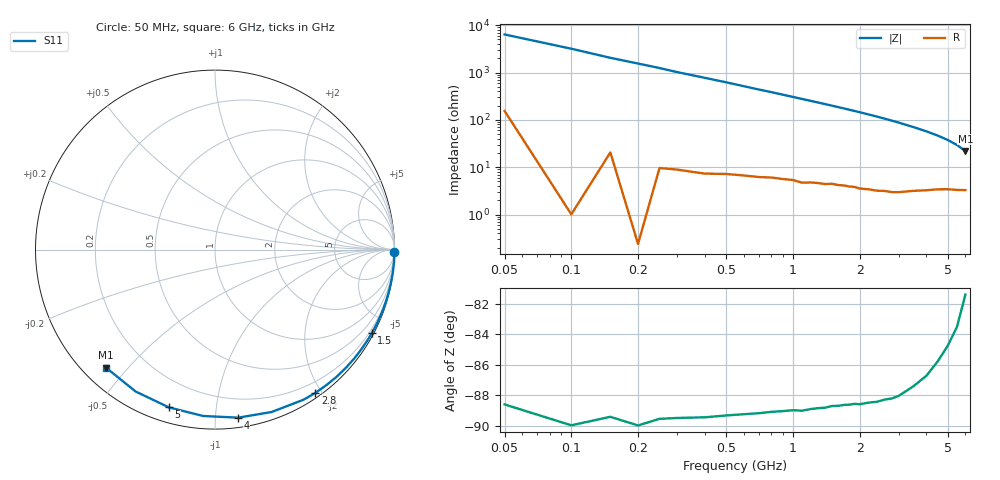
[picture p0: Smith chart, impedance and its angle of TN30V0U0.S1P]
! SIEMENS Discrete & RF Semiconductors
! BAS70-07W
! Si Schottky Diode in SOT343
! VR = 30 V
! S-Parameters:  February  1997
# GHz  S  MA  R  50
!  f  S11
! GHz  MAG  ANG
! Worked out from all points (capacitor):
!   34 points, 50 MHz to 6 GHz, reference 50 ohm
!   read as one part to ground: C = 500 fF near 50 MHz
!   lowest |Z| = 22 ohm at 6 GHz (marker M1)
!   S11 on the Smith chart (normalised r, x): 50 MHz: open; 1.5 GHz: 0.09, -3.99; 2.8 GHz: 0.06, -1.92; 4 GHz: 0.07, -1.14; 5 GHz: 0.07, -0.75; 6 GHz: 0.07, -0.44
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0.05  0.9996 -0.9
0.2  1 -3.7
0.25  0.9994 -4.6
0.3  0.9991 -5.6
0.4  0.9988 -7.4
0.6  0.9975 -11.1
0.7  0.9968 -13.0
0.8  0.996 -14.8
0.9  0.9953 -16.7
1.1  0.994 -20.5
1.3  0.9918 -24.3
1.4  0.991 -26.2
1.5  0.9895 -28.1
1.6  0.9887 -30.1
1.7  0.9875 -32.0
1.8  0.9867 -34.0
2  0.9851 -38.0
2.2  0.9825 -42.1
2.4  0.9805 -46.3
2.6  0.9772 -50.6
2.8  0.9749 -55.0
3  0.9712 -59.4
3.5  0.9583 -70.8
4  0.9451 -82.2
4.5  0.9293 -94.1
5  0.9158 -106.3
5.5  0.9058 -119.2
6  0.8953 -132.8
